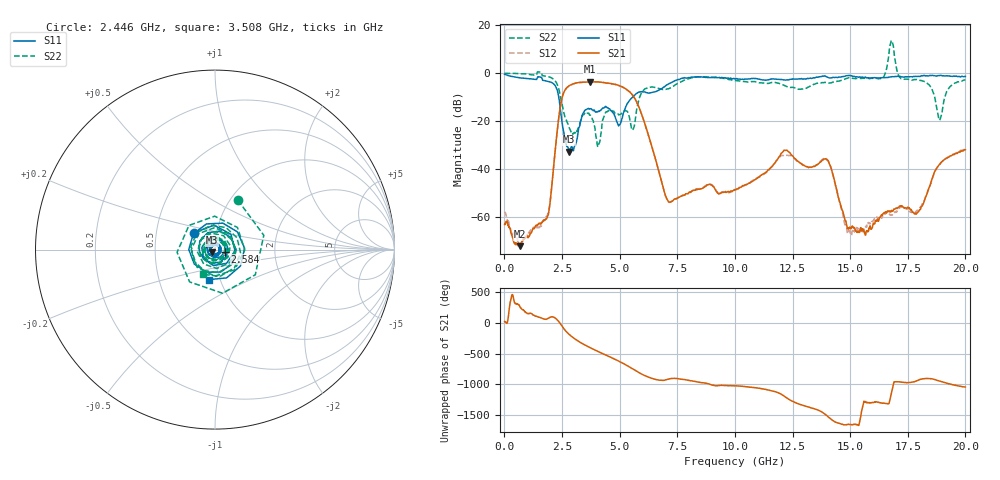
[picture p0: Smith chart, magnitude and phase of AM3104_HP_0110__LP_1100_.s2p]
!Created with skrf (http://scikit-rf.org).
# Hz S RI R 50.0
!freq ReS11 ImS11 ReS21 ImS21 ReS12 ImS12 ReS22 ImS22
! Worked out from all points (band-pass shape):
!   1601 points, 10 MHz to 20 GHz, reference 50 ohm
!   highest |S21| = -3.56 dB at 3.708 GHz (marker M1); lowest = -71.9 dB at 684.7 MHz (marker M2)
!   |S21| within 3 dB of the highest: 2.661 GHz to 5.277 GHz (2.616 GHz wide, 65.9 % of centre)
!   lowest |S11| = -32.6 dB at 2.796 GHz (marker M3), VSWR 1.05, Z = 48.2 - j1.41 ohm
!   |S11| at or under -10 dB: 2.361 GHz to 5.56 GHz (3.199 GHz wide, 80.8 % of centre)
!   |S22| runs from -30.7 to 13.6 dB; largest |S21 - S12| = 0.058
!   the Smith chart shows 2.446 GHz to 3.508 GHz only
!   S11 on the Smith chart (normalised r, x): 2.446 GHz: 0.78, +0.15; 2.584 GHz: 1.12, -0.03; 3.508 GHz: 0.88, -0.30
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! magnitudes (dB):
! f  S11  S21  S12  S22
! 10 MHz  -0.4  -62.9  -57.6  0.0
! 684.7 MHz  -1.9  -71.9  -71.1  -0.2
! 1.872 GHz  -3.3  -59.6  -58.9  -1.4
! 2.446 GHz  -16.5  -12.8  -12.9  -10.4
! 2.584 GHz  -24.8  -7.9  -7.9  -16.6
! 2.796 GHz  -32.6  -5.3  -5.3  -22.4
! 3.346 GHz  -18.6  -3.8  -3.8  -18.7
! 3.508 GHz  -15.3  -3.7  -3.7  -16.3
! 3.708 GHz  -14.8  -3.6  -3.6  -17.5
! 4.07 GHz  -15.7  -3.6  -3.7  -30.6
! 4.495 GHz  -14.4  -4.1  -4.2  -15.7
! 5.545 GHz  -10.2  -8.9  -8.9  -23.6
! 6.682 GHz  -7.2  -40.1  -40.2  -6.3
! 7.156 GHz  -4.2  -53.6  -53.7  -6.3
! 10.01 GHz  -2.4  -48.6  -48.7  -3.1
! 13.34 GHz  -2.1  -39.1  -39.1  -5.0
! 14.04 GHz  -1.7  -36.4  -36.3  -4.0
! 14.97 GHz  -0.9  -64.1  -65.6  -1.9
! 16.68 GHz  -1.6  -57.6  -58.5  7.3
! 17.95 GHz  -1.3  -57.7  -56.7  -2.7
! 18.89 GHz  -1.0  -37.8  -37.9  -19.4
! 20 GHz  -1.3  -31.8  -31.6  -2.7
